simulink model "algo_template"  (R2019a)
settings: configuration reference "configurationSettings" (kept in a data dictionary, not in this file)
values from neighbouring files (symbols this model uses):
  Value = mystruct.(myfield)    [SCDsignal_struct_to_bus.m]
undefined symbols (not defined in the file or in its folder): algo_template_fp, algo_template_tp, ProductionState, QualityTag, signal1, signal2

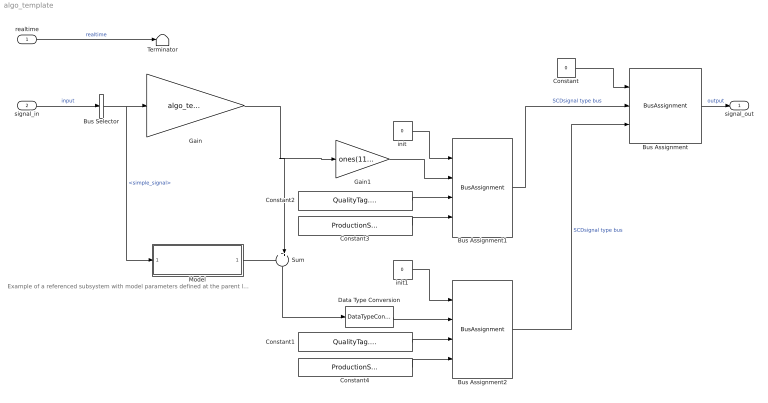
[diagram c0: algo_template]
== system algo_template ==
  note: Example of a referenced subsystem with model parameters defined at the parent level
  realtime : Inport  OutDataTypeStr=single  PortDimensions=1  SampleTime=algo_template_fp.timing.dt  Interpolate=off
  signal_in : Inport  Port=2  OutDataTypeStr=Bus: algo_template_inBus  PortDimensions=1  Interpolate=off
  Bus Assignment : BusAssignment  AssignedSignals=signal1,signal2
  Bus Assignment1 : BusAssignment  AssignedSignals=Value,QualityTag,ProductionState
  Bus Assignment2 : BusAssignment  AssignedSignals=Value,QualityTag,ProductionState
  Bus Selector : BusSelector  OutputSignals=simple_signal
  Constant : Constant  Value=0  OutDataTypeStr=Bus: algo_template_outBus
  Constant1 : Constant  Value=QualityTag.INVALID  OutDataTypeStr=Enum: QualityTag
  Constant2 : Constant  Value=QualityTag.GOOD  OutDataTypeStr=Enum: QualityTag
  Constant3 : Constant  Value=ProductionState.RUNNING  OutDataTypeStr=Enum: ProductionState
  Constant4 : Constant  Value=ProductionState.OUTDATED  OutDataTypeStr=Enum: ProductionState
  Data Type Conversion : DataTypeConversion  OutDataTypeStr=int32
  Gain : Gain  Gain=algo_template_tp.gain
  Gain1 : Gain  Gain=ones(11,1)
  Model : ModelReference  ModelNameDialog=referenced_model_example.slx  ParameterArgumentNames=TP  ParameterArgumentValues=algo_template_tp.refmodel  UsingDefaultArgumentValue=0  SimulationMode=Normal  ModelReferenceVersion=1.8
  Sum : Sum  Inputs=++|
  Terminator : Terminator
  init : Constant  Value=0  OutDataTypeStr=Bus: SCDBus_single_11_Vector
  init1 : Constant  Value=0  OutDataTypeStr=Bus: SCDBus_int32_Scalar
  signal_out : Outport  OutDataTypeStr=Bus: algo_template_outBus
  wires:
  signal_in/1 -> Bus Selector/1  "input"
  Bus Selector/1 -> Model/1, Gain/1  "<simple_signal>"
  Constant/1 -> Bus Assignment/1
  realtime/1 -> Terminator/1  "realtime"
  Bus Assignment/1 -> signal_out/1  "output"
  init/1 -> Bus Assignment1/1
  Bus Assignment1/1 -> Bus Assignment/2  "SCDsignal type bus"
  Constant2/1 -> Bus Assignment1/3
  Constant3/1 -> Bus Assignment1/4
  Gain/1 -> Sum/2, Gain1/1
  Gain1/1 -> Bus Assignment1/2
  init1/1 -> Bus Assignment2/1
  Data Type Conversion/1 -> Bus Assignment2/2
  Constant1/1 -> Bus Assignment2/3
  Constant4/1 -> Bus Assignment2/4
  Bus Assignment2/1 -> Bus Assignment/3  "SCDsignal type bus"
  Sum/1 -> Data Type Conversion/1
  Model/1 -> Sum/1
